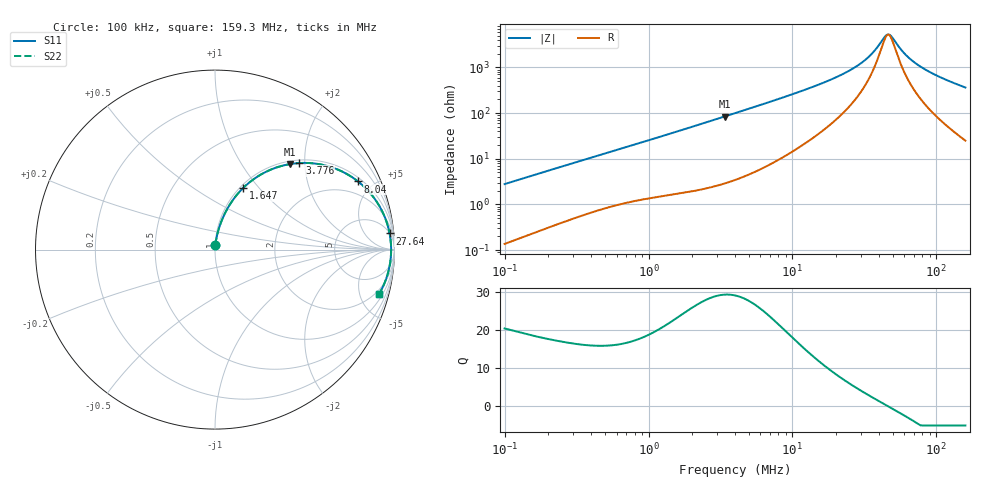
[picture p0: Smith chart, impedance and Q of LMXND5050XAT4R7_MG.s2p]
! LMXND5050XAT4R7_MG  S-PARAMETER MODEL  ( General Type )
! Model Generated by TAIYO YUDEN Corporation (http://www.ty-top.com)
! Version 1.0
! TAIYO YUDEN Control No. 191023NI43SB-FBB
! Copyright(c) 2019 TAIYO YUDEN CO.,LTD. All Rights Reserved.
! Product Description (link to TY-COMPAS)
! https://ds.yuden.co.jp/TYCOMPAS/or/detail?pn=LMXND5050XAT4R7MMG&u=M
! Products Name : Inductors
! Characteristics :
!  Inductance : 4.7 uH , SRF(min) : 31 MHz , DC Resistance(max) : 0.0455 Ohm
!  Rated Current : Saturation :3100 mA , Temp Rise : 2600 mA
!  Case Size : 4.9 x 4.9 / 0.193 x 0.193 [mm/inch] , Thickness : 3.1 / 0.122 [mm/inch]
!  (Conditions: Temperature = 25 degC , DC Bias Current/Voltage = 0A / 0V)
! External Node Assignments :
!  1  o---GGG---o  2
! GND o---------o GND
! Frequency Range : 0.1MHz  -  159.254811MHz  [ 402 STEP ]
# MHz S RI R 50
! Freq[MHz].  S11 Real  S11 Imag  S21 Real  S21 Imag  S12 Real  S12 Imag  S22 Real  S22 Imag
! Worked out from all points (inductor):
!   401 points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, 100 kHz to 159.3 MHz, reference 50 ohm
!   read as one part in series: L = 4.4 uH near 103.8 kHz
!   highest Q = 29.3 at 3.381 MHz (marker M1), where L = 3.96 uH
!   self-resonance near 46.34 MHz
!   S11 on the Smith chart (normalised r, x): 100 kHz: 1.00, +0.06; 1.647 MHz: 1.03, +0.82; 3.776 MHz: 1.06, +1.88; 8.04 MHz: 1.19, +4.09; 27.64 MHz: 5, +20; 159.3 MHz: 1.50, -7.24
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0.1  0.00213 0.0277  0.9979 -0.0277  0.9979 -0.0277  0.00213 0.0277
0.343835  0.0138 0.0898  0.9862 -0.0898  0.9862 -0.0898  0.0138 0.0898
0.655441  0.0371 0.161  0.9629 -0.161  0.9629 -0.161  0.0371 0.161
1.182227  0.0925 0.2661  0.9075 -0.2661  0.9075 -0.2661  0.0925 0.2661
1.647385  0.1553 0.3417  0.8447 -0.3417  0.8447 -0.3417  0.1553 0.3417
2.33827  0.2608 0.4212  0.7392 -0.4212  0.7392 -0.4212  0.2608 0.4212
3.380642  0.4175 0.4764  0.5825 -0.4764  0.5825 -0.4764  0.4175 0.4764
3.775988  0.4706 0.4823  0.5294 -0.4823  0.5294 -0.4823  0.4706 0.4823
4.064915  0.5065 0.483  0.4935 -0.483  0.4935 -0.483  0.5065 0.483
5.560841  0.6549 0.4569  0.3451 -0.4569  0.3451 -0.4569  0.6549 0.4569
8.039797  0.7964 0.38  0.2036 -0.38  0.2036 -0.38  0.7964 0.38
13.72135  0.9164 0.2417  0.0836 -0.2417  0.0836 -0.2417  0.9164 0.2417
20.58315  0.9579 0.1483  0.0421 -0.1483  0.0421 -0.1483  0.9579 0.1483
27.64366  0.9728 0.09  0.0272 -0.09  0.0272 -0.09  0.9728 0.09
35.12882  0.979 0.0471  0.021 -0.0471  0.021 -0.0471  0.979 0.0471
44.64076  0.9813 0.00629  0.0187 -0.00629  0.0187 -0.00629  0.9813 0.00629
47.17884  0.9814 -0.00302  0.0186 0.00302  0.0186 0.00302  0.9814 -0.00302
49.86123  0.9812 -0.0123  0.0188 0.0123  0.0188 0.0123  0.9812 -0.0123
61.06896  0.9792 -0.0469  0.0208 0.0469  0.0208 0.0469  0.9792 -0.0469
74.79595  0.9744 -0.0831  0.0256 0.0831  0.0256 0.0831  0.9744 -0.0831
104.2251  0.9585 -0.1483  0.0415 0.1483  0.0415 0.1483  0.9585 -0.1483
159.2548  0.9149 -0.2467  0.0851 0.2467  0.0851 0.2467  0.9149 -0.2467
